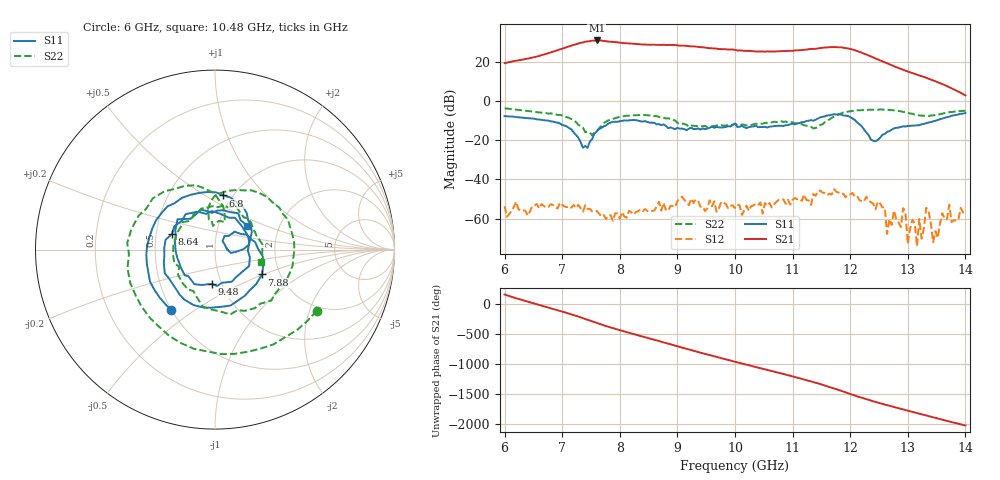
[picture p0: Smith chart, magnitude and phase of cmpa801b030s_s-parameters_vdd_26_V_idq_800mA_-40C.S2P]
!Keysight Technologies,E5071C,MY46110325,B.14.03
!Date: Tue Aug 11 10:44:42 2020
!Data & Calibration Information:
!Freq	S11:SOLT2(ON)	S21:SOLT2(ON)	S12:SOLT2(ON)	S22:SOLT2(ON)
!PortZ  Port1:50+j0  Port2:50+j0
!Above PortZ is port z conversion or system Z0 setting when saving the data.
!When reading, reference impedance value at option line is always used.
# Hz S dB R 50
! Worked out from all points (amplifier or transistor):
!   201 points, 6 GHz to 14 GHz, reference 50 ohm
!   highest |S21| = 31.1 dB at 7.6 GHz (marker M1)
!   |S21| within 3 dB of that: 7.125 GHz to 9.227 GHz (2.102 GHz wide, 25.7 % of centre)
!   unconditionally stable (mu >= 1): start of sweep to end of sweep
!   at 7.32 GHz: K = 8.21, MAG = 30.2 dB, |S12| = -54.7 dB
!   at 10 GHz: K = 11.41, MAG = 26.9 dB, |S12| = -54.7 dB
!   at 14 GHz: K = 125.18, MAG = 6.0 dB, |S12| = -56.9 dB
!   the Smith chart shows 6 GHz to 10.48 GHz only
!   S11 on the Smith chart (normalised r, x): 6 GHz: 0.50, -0.40; 6.8 GHz: 0.90, +0.60; 7.88 GHz: 1.62, -0.49; 8.64 GHz: 0.61, +0.11; 9.48 GHz: 0.90, -0.36; 10.48 GHz: 1.37, +0.38
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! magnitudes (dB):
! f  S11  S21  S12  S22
! 6 GHz  -7.6  19.5  -53.7  -3.6
! 6.8 GHz  -10.3  25.0  -52.7  -6.2
! 7.36 GHz  -23.8  30.1  -56.5  -13.5
! 7.6 GHz  -15.5  31.1  -56.2  -15.3
! 7.88 GHz  -10.6  30.3  -61.1  -9.0
! 8.64 GHz  -11.9  28.8  -53.7  -7.5
! 8.68 GHz  -11.7  28.9  -51.5  -8.1
! 9.48 GHz  -14.3  27.4  -56.2  -12.6
! 10 GHz  -11.4  26.3  -54.7  -11.5
! 10.48 GHz  -13.2  25.5  -57.5  -11.5
! 11.36 GHz  -10.0  26.8  -47.5  -13.9
! 12.68 GHz  -15.3  18.8  -60.3  -4.5
! 12.92 GHz  -12.8  16.1  -54.7  -5.5
! 13 GHz  -12.7  15.2  -72.9  -6.0
! 13.08 GHz  -12.5  14.4  -60.6  -6.4
! 13.16 GHz  -12.3  13.6  -74.1  -7.0
! 13.2 GHz  -12.3  13.2  -60.2  -7.3
! 13.24 GHz  -11.8  12.8  -70.3  -7.4
! 13.32 GHz  -11.2  12.0  -54.5  -7.5
! 13.44 GHz  -10.3  10.7  -72.1  -7.2
! 13.72 GHz  -7.9  7.2  -53.0  -5.6
! 14 GHz  -6.1  3.0  -56.9  -4.8
